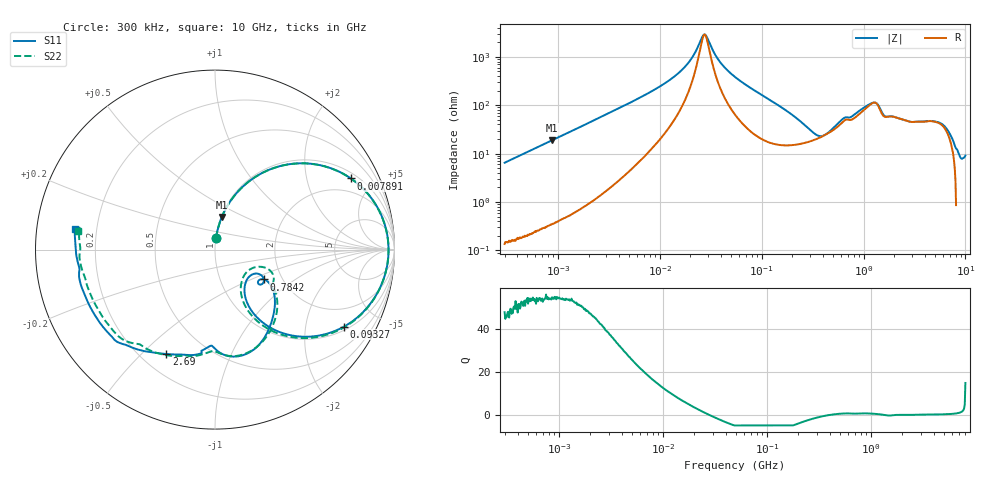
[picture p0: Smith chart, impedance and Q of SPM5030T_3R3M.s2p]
! S-Parameter Data Generated by TDK Corporation
! Copyright(C) 2019 TDK Corporation.
! All Rights Reserved.
! TDK P/N: SPM5030T-3R3M (Inductor)
! Property: L=3.3uH at 100kHz
! Size(LxWxT): 5.2x5x3mm
! Model Type: s2p (Touchstone File Format Version 1.0)
! Frequency: DC=Yes Start=0.3MHz Stop=10000MHz 802points Log-sweep
! Model Generated on Sep. 23, 2019
! Port Assignments:
!  1 ---@@@--- 2
! Applicable Conditions:
!  Temperature = 25 degC
!  DC Bias Current = 0 A
!  Small Signal Operation
! Terms and conditions regarding TDK Simulation Models
! (1)This simulation model is being provided solely for informational purposes. Please refer to the specifications of the products in terms of detailed characteristics of such products.
! (2)In no event shall TDK Corporation of any of its subsidiaries be liable for any loss or damage arising, directly or indirectly,
!  From any information contained in this simulation model, including, but not limited to loss or damages arising from any inaccuracies, omissions or errors in connection with such information.
! (3)Any and all copyrights on this simulation model are owned by TDK Corporation.
!  Duplication or redistribution of this simulation model without prior written permission from TDK Corporation is prohibited.
! (4)This simulation model is subject to any modification or change without any prior notice.
! (5)Neither TDK Corporation nor any of its subsidiaries shall make any warranty, express or implied,
!  Including but not limited to the correctness, implied warranties of merchantability and fitness for a particular purpose with respect to this simulation models.
! (6)The use of this simulation model shall be deemed to have consented to the terms and conditions hereof.
# Hz S MA R 50
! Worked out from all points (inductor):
!   801 points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, 300 kHz to 10 GHz, reference 50 ohm
!   read as one part in series: L = 3.43 uH near 318.3 kHz
!   highest Q = 54.1 at 881.6 kHz (marker M1), where L = 3.42 uH
!   self-resonance near 27.57 MHz
!   S11 on the Smith chart (normalised r, x): 300 kHz: 1.00, +0.13; 7.891 MHz: 1.25, +3.67; 93.27 MHz: 1.14, -3.26; 784.2 MHz: 1.61, -0.60; 2.69 GHz: 0.30, -0.60; 10 GHz: 0.12, +0.07
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300000  0.06431 85.0  0.9964 -3.7  0.9967 -3.7  0.06426 85.1
881608  0.1854 78.2  0.9792 -10.7  0.9793 -10.7  0.1853 78.2
1713600  0.343 68.7  0.9324 -20.1  0.9325 -20.1  0.343 68.7
4001173  0.6461 47.8  0.7426 -40.4  0.7426 -40.4  0.6461 47.7
7890546  0.8549 27.6  0.4694 -58.9  0.4694 -58.9  0.8548 27.6
9671944  0.8946 22.1  0.3835 -63.5  0.3835 -63.5  0.8944 22.0
1.786051e7  0.9578 7.7  0.1502 -70.3  0.1503 -70.3  0.9577 7.6
2.725275e7  0.9669 -0.9  0.03348 -7.5  0.03348 -7.5  0.9666 -1.1
3.904515e7  0.9576 -8.3  0.1219 64.5  0.122 64.5  0.9571 -8.6
5.477226e7  0.9318 -16.0  0.241 64.3  0.241 64.3  0.9311 -16.4
9.327145e7  0.8371 -30.8  0.4571 52.0  0.4572 52.0  0.8359 -31.5
1.653189e8  0.6234 -49.4  0.6871 30.5  0.6872 30.5  0.6204 -50.7
3.126428e8  0.3222 -57.9  0.8082 2.1  0.8083 2.1  0.3104 -60.9
4.687561e8  0.2456 -35.7  0.7705 -16.7  0.7706 -16.7  0.2167 -34.9
7.84152e8  0.319 -31.4  0.6293 -35.3  0.6293 -35.3  0.3829 -32.2
1.212691e9  0.5302 -55.1  0.4026 -45.8  0.4025 -45.8  0.5686 -60.6
1.43752e9  0.6088 -75.6  0.4027 -34.0  0.4027 -34.0  0.6012 -80.9
1.767019e9  0.5359 -92.5  0.4598 -47.6  0.4598 -47.6  0.5776 -94.6
2.69003e9  0.6421 -115.0  0.3828 -67.5  0.3828 -67.5  0.6674 -122.5
6.091595e9  0.7563 -143.9  0.2197 -108.4  0.2197 -108.4  0.7301 -149.4
8.770142e9  0.7727 -177.3  0.1586 -139.4  0.1587 -139.3  0.7611 174.4
1e10  0.7879 171.8  0.1317 -146.6  0.1318 -146.6  0.7686 172.2
